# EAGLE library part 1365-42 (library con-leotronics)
DUAL ROW STRAIGHT HEADER 1364 SERIES. 1.27mm x 1.27mm. Without Fixing Post. SMT Source: http://www.leotronics.co.uk/Conexcon/Data%20Sheets/sec.%20A/1364ing.pdf
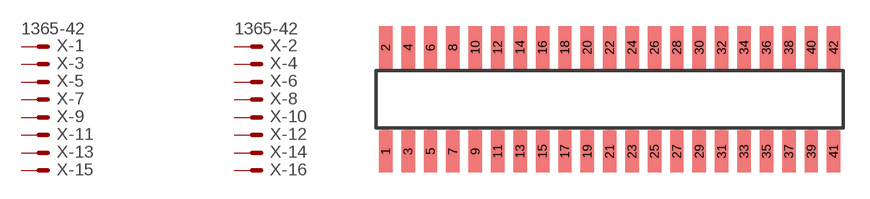
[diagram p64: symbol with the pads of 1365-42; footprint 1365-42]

Designator prefix X; gates -1=MVAL -2=MVAL -3=M -4=M -5=M -6=M -7=M -8=M -9=M -10=M -11=M -12=M -13=M -14=M -15=M -16=M -17=M -18=M -19=M -20=M -21=M -22=M -23=M -24=M -25=M -26=M -27=M -28=M -29=M -30=M -31=M -32=M -33=M -34=M -35=M -36=M -37=M -38=M -39=M -40=M -41=M -42=M

## 1365-42 (OC_FARNELL: unknown; OC_NEWARK: unknown)  [1365-42]
1  -1:S  pas
2  -2:S  pas
3  -3:S  pas
4  -4:S  pas
5  -5:S  pas
6  -6:S  pas
7  -7:S  pas
8  -8:S  pas
9  -9:S  pas
10  -10:S  pas
11  -11:S  pas
12  -12:S  pas
13  -13:S  pas
14  -14:S  pas
15  -15:S  pas
16  -16:S  pas
17  -17:S  pas
18  -18:S  pas
19  -19:S  pas
20  -20:S  pas
21  -21:S  pas
22  -22:S  pas
23  -23:S  pas
24  -24:S  pas
25  -25:S  pas
26  -26:S  pas
27  -27:S  pas
28  -28:S  pas
29  -29:S  pas
30  -30:S  pas
31  -31:S  pas
32  -32:S  pas
33  -33:S  pas
34  -34:S  pas
35  -35:S  pas
36  -36:S  pas
37  -37:S  pas
38  -38:S  pas
39  -39:S  pas
40  -40:S  pas
41  -41:S  pas
42  -42:S  pas

## Footprint 1365-42 (pad centres in mm)
DUAL ROW STRAIGHT HEADER 1364 SERIES. 1.27mm x 1.27mm. Without Fixing Post. SMT Source: http://www.leotronics.co.uk/Conexcon/Data%20Sheets/sec.%20A/1364ing.pdf
smd 0.76 x 2.4: 1 -12.7,-2.95; 2 -12.7,2.95; 3 -11.43,-2.95; 4 -11.43,2.95; 5 -10.16,-2.95; 6 -10.16,2.95; 7 -8.89,-2.95; 8 -8.89,2.95; 9 -7.62,-2.95; 10 -7.62,2.95; 11 -6.35,-2.95; 12 -6.35,2.95; 13 -5.08,-2.95; 14 -5.08,2.95; 15 -3.81,-2.95; 16 -3.81,2.95; 17 -2.54,-2.95; 18 -2.54,2.95; 19 -1.27,-2.95; 20 -1.27,2.95; 21 0,-2.95; 22 0,2.95; 23 1.27,-2.95; 24 1.27,2.95; 25 2.54,-2.95; 26 2.54,2.95; 27 3.81,-2.95; 28 3.81,2.95; 29 5.08,-2.95; 30 5.08,2.95; 31 6.35,-2.95; 32 6.35,2.95; 33 7.62,-2.95; 34 7.62,2.95; 35 8.89,-2.95; 36 8.89,2.95; 37 10.16,-2.95; 38 10.16,2.95; 39 11.43,-2.95; 40 11.43,2.95; 41 12.7,-2.95; 42 12.7,2.95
